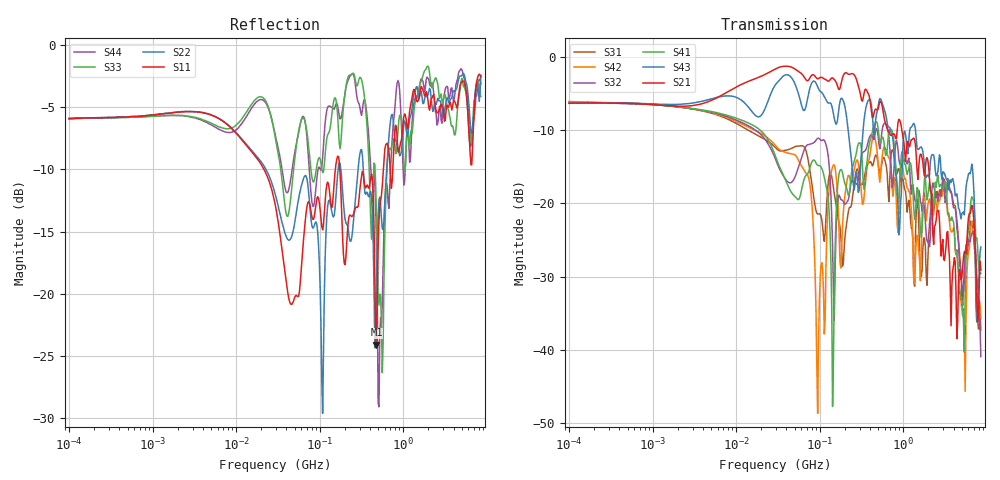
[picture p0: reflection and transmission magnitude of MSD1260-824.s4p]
# MHz S MA R 50
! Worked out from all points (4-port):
!   498 points, 100 kHz to 8.5 GHz, reference 50 ohm
!   strongest paths, dB at 100 kHz, 1.698 MHz, 29.49 MHz, 500.7 MHz, 8.5 GHz:
!     S21: -6.3, -6.7, -1.7, -7.1, -29.1
!     S43: -6.3, -6.5, -3.8, -6.7, -26.0
!     S41: -6.4, -6.8, -13.6, -9.8, -29.5
!     S32: -6.3, -6.8, -13.9, -10.9, -40.9
!     S42: -6.1, -6.8, -12.1, -14.4, -35.7
!     S31: -6.1, -6.7, -12.4, -14.6, -37.3
!   lowest |S11| = -24.1 dB at 478.3 MHz (marker M1), VSWR 1.13, Z = 56.5 - j1.4 ohm
!   |S11| at or under -10 dB: 21.51 MHz to 153.9 MHz (132.4 MHz wide, 151 % of centre); 173.9 MHz to 578.1 MHz (404.1 MHz wide, 107 % of centre); 696.8 MHz to 749.2 MHz (52.43 MHz wide, 7.25 % of centre)
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0.1  0.5058 5.6  0.4823 5.8  0.4941 -7.0  0.4812 -175.6
     0.4823 5.8  0.5058 5.6  0.4815 -175.4  0.4944 -7.0
     0.4941 -7.0  0.4815 -175.4  0.5057 5.6  0.4825 5.7
     0.4812 -175.6  0.4944 -7.0  0.4825 5.7  0.5052 5.7
51.0163  0.09805 -3.7  0.8211 -13.8  0.244 34.1  0.1107 -164.4
         0.8211 -13.8  0.1993 -2.2  0.153 -159.0  0.2128 49.9
         0.244 34.1  0.153 -159.0  0.3636 16.5  0.6445 -26.0
         0.1107 -164.4  0.2128 49.9  0.6445 -26.0  0.3804 7.4
94.51579  0.2455 2.4  0.707 -20.8  0.08455 -155.2  0.1815 34.8
          0.707 -20.8  0.1775 -44.9  0.2777 45.2  0.003693 145.5
          0.08455 -155.2  0.2777 45.2  0.3397 1.5  0.6241 -34.0
          0.1815 34.8  0.003693 145.5  0.6241 -34.0  0.3099 11.2
142.5721  0.2305 3.5  0.7167 -29.8  0.1405 29.8  0.004108 -92.0
          0.7167 -29.8  0.2066 4.5  0.05096 -93.7  0.1771 45.3
          0.1405 29.8  0.05096 -93.7  0.5572 7.0  0.4389 -52.2
          0.004108 -92.0  0.1771 45.3  0.4389 -52.2  0.5575 -4.1
478.3074  0.06256 -11.4  0.4361 -84.3  0.2124 -37.5  0.3603 -34.3
          0.4361 -84.3  0.1048 11.8  0.323 -30.1  0.2436 -51.4
          0.2124 -37.5  0.323 -30.1  0.2058 -122.2  0.4049 -50.4
          0.3603 -34.3  0.2436 -51.4  0.4049 -50.4  0.1568 -144.6
6034.534  0.4824 -155.6  0.07999 76.5  0.05562 149.5  0.06518 -165.6
          0.07999 76.5  0.603 -152.5  0.05524 156.8  0.04654 -170.4
          0.05562 149.5  0.05524 156.8  0.5671 -141.3  0.1581 99.9
          0.06518 -165.6  0.04654 -170.4  0.1581 99.9  0.483 179.4
8500  0.7437 -54.3  0.03513 -105.6  0.01364 -117.1  0.03331 -116.9
      0.03513 -105.6  0.7547 -41.2  0.008991 34.5  0.01637 -80.4
      0.01364 -117.1  0.008991 34.5  0.6194 -44.1  0.05034 -43.5
      0.03331 -116.9  0.01637 -80.4  0.05034 -43.5  0.6973 -54.5
